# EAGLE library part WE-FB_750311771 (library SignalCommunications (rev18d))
WE-FB Flyback Transformer suitable for LT3573/ LT3574/ LT3575/ LT3748 Characteristics easy design in solution less external components needed small board space low cost no optocoupler needed! long term reliability voltage control no aging same external parts for different output voltages easy design of custom power supply due to standard circuit and change of transformers and two components for feedback loop Isolation voltage up to 2.5 kV Applications Isolated power design Sensor interfaces Isolated telecom converters Power over Ethernet Details see: http://katalog.we-online.de/en/pbs/WE-FB_Linear? Updated 2015-04-03 2015 (C) Wurth Elektronik
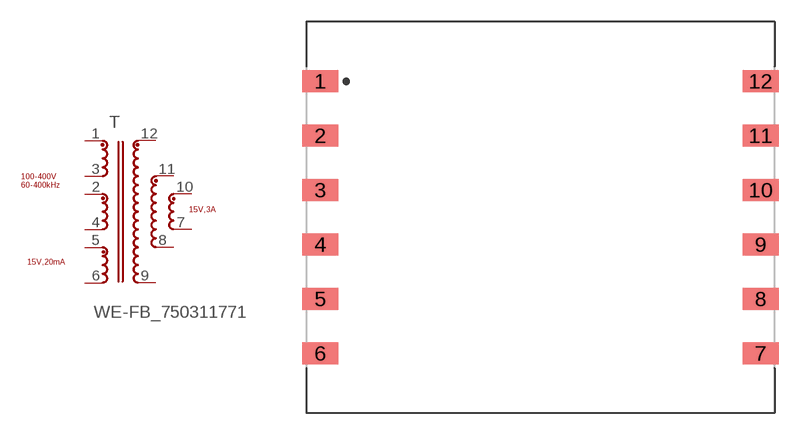
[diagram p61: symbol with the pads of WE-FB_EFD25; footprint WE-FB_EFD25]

Designator prefix T

## WE-FB_750311771  [WE-FB_EFD25]
1  1  pas
2  11  pas
3  12  pas
4  10  pas
5  9  pas
6  8  pas
7  5  pas
8  6  pas
9  7  pas
10  4  pas
11  3  pas
12  2  pas

## Footprint WE-FB_EFD25 (pad centres in mm)
smd 2.5 x 1.52: 1 -15.19,9.4; 2 -15.19,5.64; 3 -15.19,1.88; 4 -15.19,-1.88; 5 -15.19,-5.64; 6 -15.19,-9.4; 7 15.19,-9.4; 8 15.19,-5.64; 9 15.19,-1.88; 10 15.19,1.88; 11 15.19,5.64; 12 15.19,9.4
